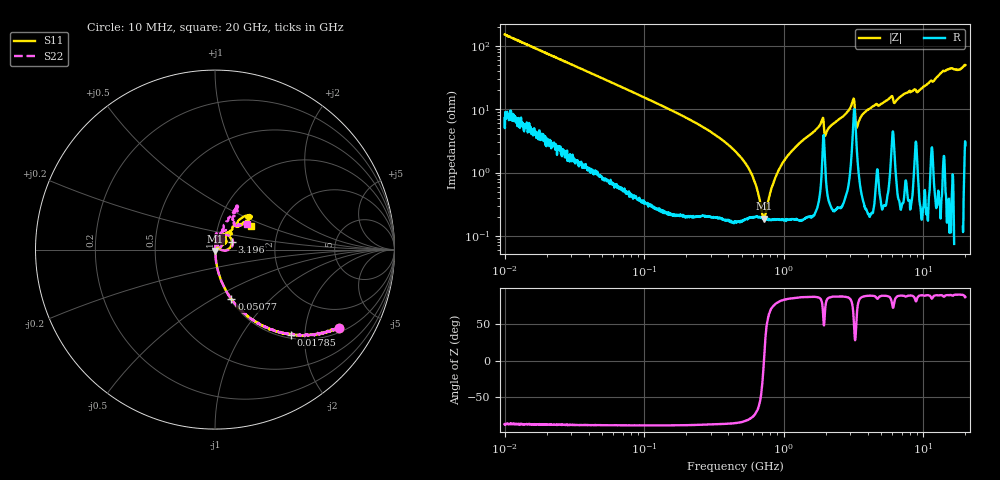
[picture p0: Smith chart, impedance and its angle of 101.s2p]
!Keysight Technologies,P5008B,MY61100088,A.16.20.02
!Date: Friday, August 30, 2024 14:37:15
!Correction: S11(C  2-Port  )
!S21(C  2-Port  )
!S12(C  2-Port  )
!S22(C  2-Port  )
!S2P File: Measurements: S11, S21, S12, S22:Log Frequency Sweep
# Hz S  MA  R 50
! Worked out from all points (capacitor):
!   1601 points, 10 MHz to 20 GHz, reference 50 ohm
!   read as one part in series: C = 104 pF near 10.39 MHz
!   lowest |Z| = 186 mohm at 722.6 MHz (marker M1)
!   series resonance near 720.8 MHz, so ESL is about 470 pH
!   S11 on the Smith chart (normalised r, x): 10 MHz: 1.14, -3.06; 17.85 MHz: 1.07, -1.70; 50.77 MHz: 1.02, -0.61; 3.196 GHz: 1.20, +0.10; 20 GHz: 1.43, +0.41
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1e7  0.8204 -32.3  0.5352 55.0  0.5352 55.0  0.8199 -32.3
1.785268e7  0.6359 -48.3  0.7473 39.4  0.7472 39.4  0.6358 -48.3
3.555162e7  0.3959 -64.9  0.906 23.3  0.906 23.3  0.3959 -64.9
5.07686e7  0.2911 -71.6  0.9492 16.9  0.9492 16.8  0.291 -71.7
1.263918e8  0.1216 -82.0  0.99 6.8  0.9897 6.8  0.1216 -82.2
4.472136e8  0.02659 -84.6  0.9978 1.0  0.9976 1.0  0.02649 -87.3
7.225909e8  0.007233 -75.0  0.9981 -0.4  0.9978 -0.4  0.007191 -79.3
8.86355e8  0.002532 -4.6  0.9981 -1.0  0.9979 -1.0  0.0006477 -7.8
1.051673e9  0.007945 68.1  0.9981 -1.6  0.9978 -1.6  0.007471 84.8
1.589917e9  0.02641 81.3  0.9976 -3.3  0.9973 -3.3  0.02608 84.0
1.859765e9  0.04582 73.0  0.9908 -4.6  0.9906 -4.7  0.04421 76.8
2.035438e9  0.02486 72.4  0.9945 -3.7  0.9944 -3.7  0.02378 75.5
3.091822e9  0.09086 66.7  0.9695 -8.9  0.9693 -9.0  0.09202 60.7
3.196366e9  0.1042 24.3  0.9067 -7.1  0.9064 -7.2  0.1093 22.0
3.432446e9  0.0238 71.7  0.9901 -5.8  0.9898 -5.8  0.02634 49.0
3.902191e9  0.05128 86.4  0.9965 -7.9  0.9962 -8.0  0.05132 71.5
5.652411e9  0.07089 72.8  0.9927 -12.7  0.9927 -12.8  0.07376 71.2
6.335038e9  0.05148 53.0  0.9913 -12.5  0.991 -12.6  0.04942 75.2
7.697294e9  0.0868 55.4  0.995 -16.6  0.9947 -16.7  0.08181 83.2
9.220141e9  0.05903 47.9  0.995 -19.3  0.9947 -19.5  0.05541 75.1
1.367661e10  0.2459 48.7  0.973 -31.5  0.9728 -31.7  0.2397 63.1
2e10  0.2406 33.6  0.9477 -47.0  0.9477 -47.3  0.2258 38.6
